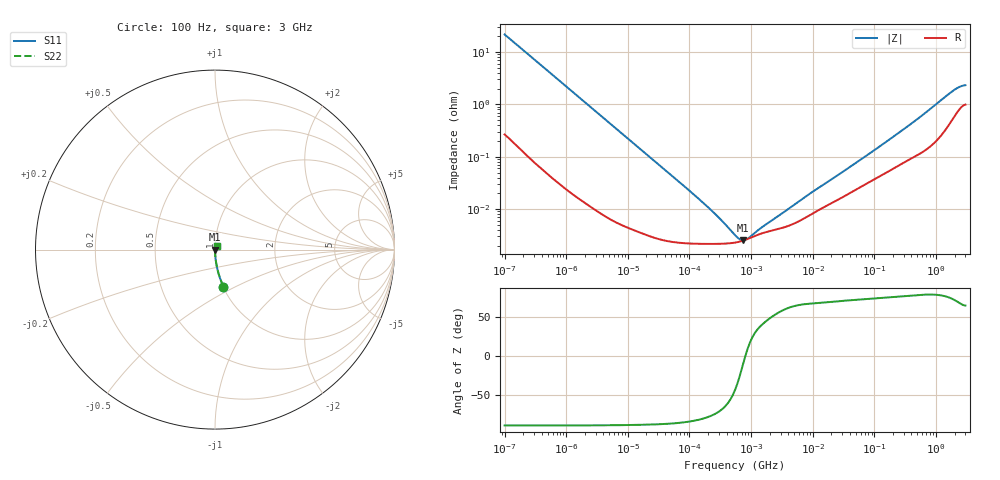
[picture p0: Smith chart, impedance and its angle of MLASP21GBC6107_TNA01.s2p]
! MLASP21GBC6107_TNA01  S-PARAMETER MODEL  ( Standard Model )
! Model Generated by TAIYO YUDEN Corporation (http://www.ty-top.com)
! Version 1.0
! TAIYO YUDEN Control No. 250116
! Copyright(c) 2025 TAIYO YUDEN CO.,LTD. All Rights Reserved.
! Product Description (link to TY-COMPAS)
! https://ds.yuden.co.jp/TYCOMPAS/or/detail?pn=MLASP21GBC6107MTNA01&u=M
! Products Name : Multilayer Ceramic Capacitors
! Characteristics :
!  Capacitance : 100 [uF] , Rated Voltage : 2.5 [V] , TCC : X6S
!  Case Size : 2.0 x 1.25 / 0.079 x 0.049 [mm/inch] , Thickness : 1.25 / 0.049 [mm/inch]
!  (Conditions: Temperature = 25 [degC] , DC Bias Voltage = 0 [V])
! External Node Assignments :
!  1  o---| |---o  2
! GND o---------o GND
! Frequency Range : 100Hz  -  3GHz  [ 401 STEP ]
# MHZ S RI R 50
! Freq[MHz].  S11 Real  S11 Imag  S21 Real  S21 Imag  S12 Real  S12 Imag  S22 Real  S22 Imag
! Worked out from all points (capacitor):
!   401 points, 100 Hz to 3 GHz, reference 50 ohm
!   read as one part in series: C = 73.1 uF near 109 Hz
!   lowest |Z| = 2.54 mohm at 740.3 kHz (marker M1)
!   series resonance near 806.9 kHz, so ESL is about 530 pH
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0.0001  0.0473 -0.2063  0.9527 0.2063  0.9527 0.2063  0.0473 -0.2063
0.000114  0.0373 -0.1835  0.9627 0.1835  0.9627 0.1835  0.0373 -0.1835
0.000199  0.0131 -0.1081  0.9869 0.1081  0.9869 0.1081  0.0131 -0.1081
0.000348  0.0046 -0.0626  0.9954 0.0626  0.9954 0.0626  0.0046 -0.0626
0.000724  0.00124 -0.0304  0.9988 0.0304  0.9988 0.0304  0.00124 -0.0304
0.001788  0.000297 -0.0124  0.9997 0.0124  0.9997 0.0124  0.000297 -0.0124
0.031977  2.71e-05 -0.000705  1 0.000705  1 0.000705  2.71e-05 -0.000705
0.097915  2.21e-05 -0.000228  1 0.000228  1 0.000228  2.21e-05 -0.000228
0.194955  2.16e-05 -0.00011  1 0.00011  1 0.00011  2.16e-05 -0.00011
0.21248  2.16e-05 -9.93e-05  1 9.93e-05  1 9.93e-05  2.16e-05 -9.93e-05
0.241767  2.16e-05 -8.54e-05  1 8.54e-05  1 8.54e-05  2.16e-05 -8.54e-05
0.547723  2.29e-05 -2.2e-05  1 2.2e-05  1 2.2e-05  2.29e-05 -2.2e-05
0.740304  2.49e-05 -4.63e-06  1 4.63e-06  1 4.63e-06  2.49e-05 -4.63e-06
3.79959  4.66e-05 8.4e-05  1 -8.4e-05  1 -8.4e-05  4.66e-05 8.4e-05
4.323298  4.93e-05 9.52e-05  1 -9.52e-05  1 -9.52e-05  4.93e-05 9.52e-05
9.794414  8.13e-05 0.000195  0.9999 -0.000195  0.9999 -0.000195  8.13e-05 0.000195
35.62563  0.000187 0.00055  0.9998 -0.00055  0.9998 -0.00055  0.000187 0.00055
175.1444  0.000541 0.00206  0.9995 -0.00206  0.9995 -0.00206  0.000541 0.00206
513.708  0.00112 0.00527  0.9989 -0.00527  0.9989 -0.00527  0.00112 0.00527
1868.531  0.00551 0.0171  0.9945 -0.0171  0.9945 -0.0171  0.00551 0.0171
2419.119  0.00849 0.0198  0.9915 -0.0198  0.9915 -0.0198  0.00849 0.0198
3000  0.0102 0.0207  0.9898 -0.0207  0.9898 -0.0207  0.0102 0.0207
